PROGRAM P_Prog1
VAR

	fbKL6401 		: FB_LON_KL6401;

	fbREAD_001		: FB_READ_001_SNVT_amp;
	fbSEND_001		: FB_SEND_001_SNVT_amp;

	fbREAD_002		: FB_READ_002_SNVT_amp_mil;
	fbSEND_002		: FB_SEND_002_SNVT_amp_mil;

	fbREAD_003		: FB_READ_003_SNVT_angle;
	fbSEND_003		: FB_SEND_003_SNVT_angle;

	fbREAD_004		: FB_READ_004_SNVT_angle_vel;
	fbSEND_004		: FB_SEND_004_SNVT_angle_vel;

	fbREAD_005		: FB_READ_005_SNVT_btu_kilo;
	fbSEND_005		: FB_SEND_005_SNVT_btu_kilo;

	fbREAD_006		: FB_READ_006_SNVT_btu_mega;
	fbSEND_006		: FB_SEND_006_SNVT_btu_mega;

	fbREAD_007		: FB_READ_007_SNVT_char_ascii;
	fbSEND_007		: FB_SEND_007_SNVT_char_ascii;

	fbREAD_008		: FB_READ_008_SNVT_count;
	fbSEND_008		: FB_SEND_008_SNVT_count;

	fbREAD_009		: FB_READ_009_SNVT_count_inc;
	fbSEND_009		: FB_SEND_009_SNVT_count_inc;
(*
	fbREAD_010		: FB_READ_011_SNVT_date_day;
	fbSEND_010		: FB_SEND_002_SNVT_amp_mil;
*)

	fbREAD_011		: FB_READ_011_SNVT_date_day;
	fbSEND_011		: FB_SEND_011_SNVT_date_day;

(*
	fbREAD_012		: FB_READ_01;
	fbSEND_012		: FB_SEND_002_SNVT_amp_mil;
*)

	fbREAD_013		: FB_READ_013_SNVT_elec_kwh;
	fbSEND_013		: FB_SEND_013_SNVT_elec_kwh;

	fbREAD_014		: FB_READ_014_SNVT_elec_whr;
	fbSEND_014		: FB_SEND_014_SNVT_elec_whr;

	fbREAD_015		: FB_READ_015_SNVT_flow;
	fbSEND_015		: FB_SEND_015_SNVT_flow;

	fbREAD_016		: FB_READ_016_SNVT_flow_mil;
	fbSEND_016		: FB_SEND_016_SNVT_flow_mil;

	fbREAD_017		: FB_READ_017_SNVT_length;
	fbSEND_017		: FB_SEND_017_SNVT_length;

	fbREAD_018		: FB_READ_018_SNVT_length_kilo;
	fbSEND_018		: FB_SEND_018_SNVT_length_kilo;

	fbREAD_019		: FB_READ_019_SNVT_length_micr;
	fbSEND_019		: FB_SEND_019_SNVT_length_micr;

	fbREAD_020		: FB_READ_020_SNVT_length_mil;
	fbSEND_020		: FB_SEND_020_SNVT_length_mil;

	fbREAD_021		: FB_READ_021_SNVT_lev_cont;
	fbSEND_021		: FB_SEND_021_SNVT_lev_cont;
(*
	fbREAD_022		: FB_READ_022;
	fbSEND_022		: FB_SEND_002_SNVT_amp_mil;
*)
	fbREAD_023		: FB_READ_023_SNVT_mass;
	fbSEND_023		: FB_SEND_023_SNVT_mass;

	fbREAD_024		: FB_READ_024_SNVT_mass_kilo;
	fbSEND_024		: FB_SEND_024_SNVT_mass_kilo;

	fbREAD_025		: FB_READ_025_SNVT_mass_mega;
	fbSEND_025		: FB_SEND_025_SNVT_mass_mega;

	fbREAD_026		: FB_READ_026_SNVT_mass_mil;
	fbSEND_026		: FB_SEND_026_SNVT_mass_mil;

	fbREAD_027		: FB_READ_027_SNVT_power;
	fbSEND_027		: FB_SEND_027_SNVT_power;

	fbREAD_028		: FB_READ_028_SNVT_power_kilo;
	fbSEND_028		: FB_SEND_028_SNVT_power_kilo;

	fbREAD_029		: FB_READ_029_SNVT_ppm;
	fbSEND_029		: FB_SEND_029_SNVT_ppm;

	fbREAD_030		: FB_READ_030_SNVT_press;
	fbSEND_030		: FB_SEND_030_SNVT_press;

	fbREAD_031		: FB_READ_031_SNVT_res;
	fbSEND_031		: FB_SEND_031_SNVT_res;

END_VAR

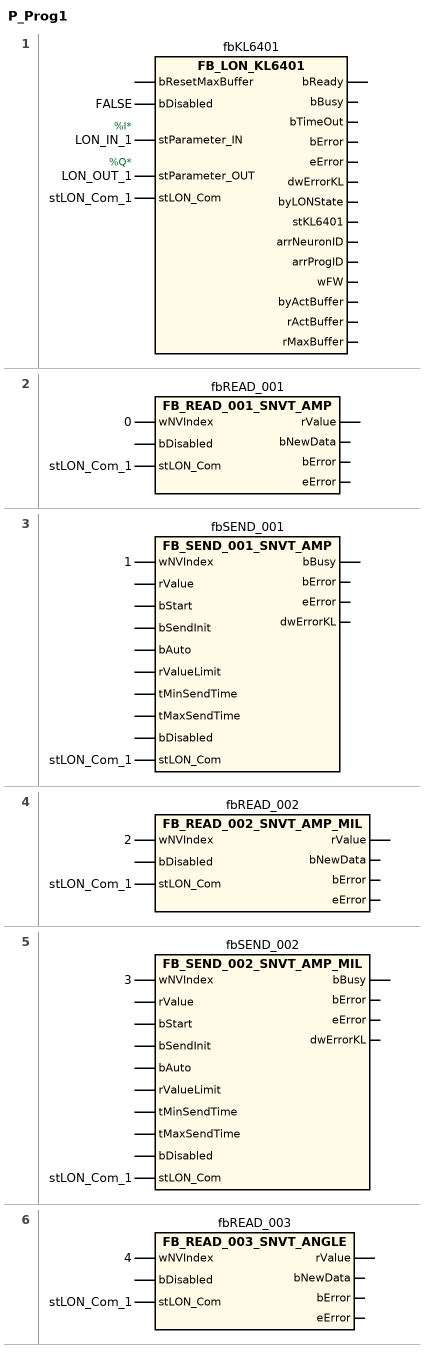
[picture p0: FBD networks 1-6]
// NETWORK 1
//   LON_IN_1: AT %I*
//   LON_OUT_1: AT %Q*
fbKL6401(
    bDisabled := FALSE,
    stParameter_IN := LON_IN_1,
    stParameter_OUT := LON_OUT_1,
    stLON_Com := stLON_Com_1); // FB_LON_KL6401

// NETWORK 2
fbREAD_001(wNVIndex := 0, stLON_Com := stLON_Com_1); // FB_READ_001_SNVT_AMP

// NETWORK 3
fbSEND_001(wNVIndex := 1, stLON_Com := stLON_Com_1); // FB_SEND_001_SNVT_AMP

// NETWORK 4
fbREAD_002(wNVIndex := 2, stLON_Com := stLON_Com_1); // FB_READ_002_SNVT_AMP_MIL

// NETWORK 5
fbSEND_002(wNVIndex := 3, stLON_Com := stLON_Com_1); // FB_SEND_002_SNVT_AMP_MIL

// NETWORK 6
fbREAD_003(wNVIndex := 4, stLON_Com := stLON_Com_1); // FB_READ_003_SNVT_ANGLE

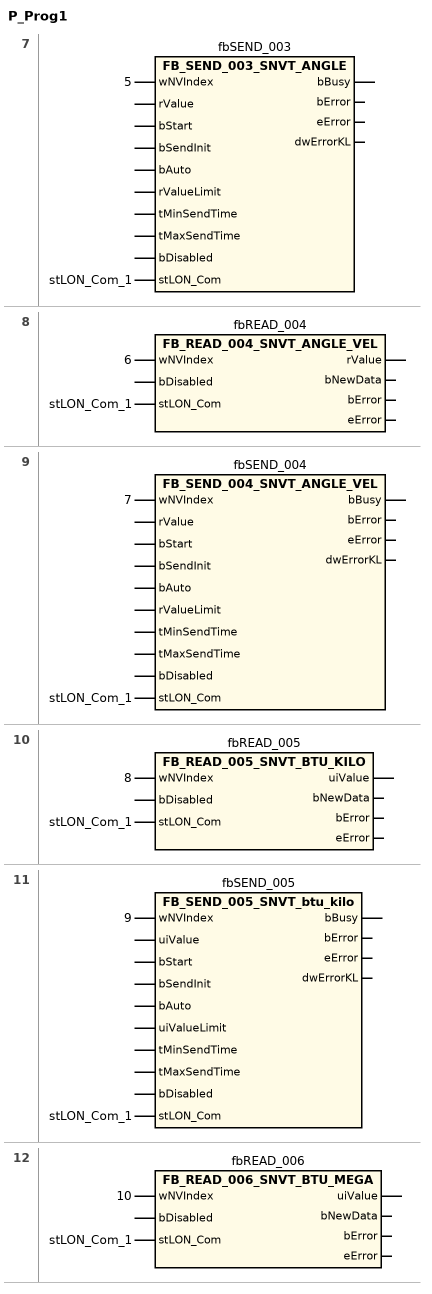
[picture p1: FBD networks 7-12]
// NETWORK 7
fbSEND_003(wNVIndex := 5, stLON_Com := stLON_Com_1); // FB_SEND_003_SNVT_ANGLE

// NETWORK 8
fbREAD_004(wNVIndex := 6, stLON_Com := stLON_Com_1); // FB_READ_004_SNVT_ANGLE_VEL

// NETWORK 9
fbSEND_004(wNVIndex := 7, stLON_Com := stLON_Com_1); // FB_SEND_004_SNVT_ANGLE_VEL

// NETWORK 10
fbREAD_005(wNVIndex := 8, stLON_Com := stLON_Com_1); // FB_READ_005_SNVT_BTU_KILO

// NETWORK 11
fbSEND_005(wNVIndex := 9, stLON_Com := stLON_Com_1); // FB_SEND_005_SNVT_btu_kilo

// NETWORK 12
fbREAD_006(wNVIndex := 10, stLON_Com := stLON_Com_1); // FB_READ_006_SNVT_BTU_MEGA

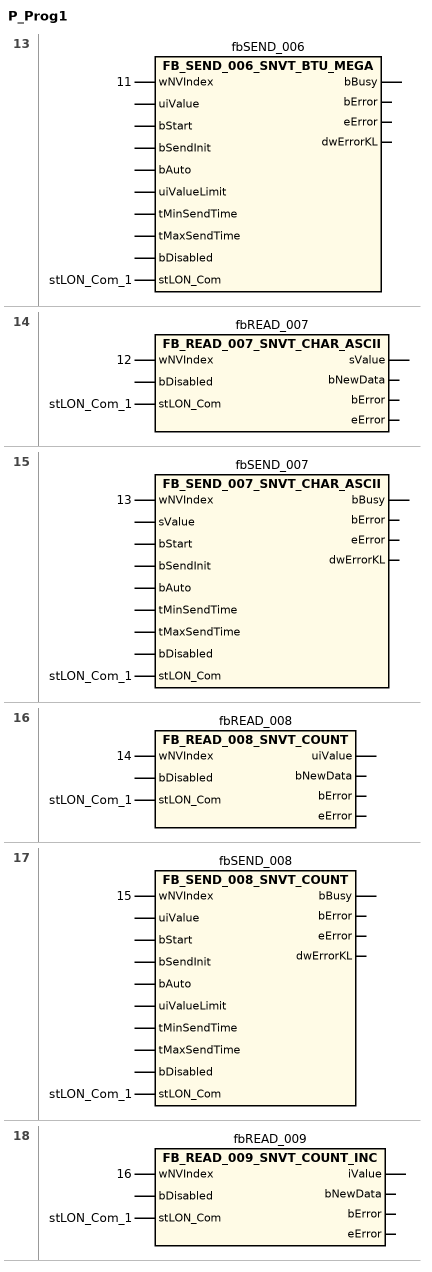
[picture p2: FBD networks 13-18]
// NETWORK 13
fbSEND_006(wNVIndex := 11, stLON_Com := stLON_Com_1); // FB_SEND_006_SNVT_BTU_MEGA

// NETWORK 14
fbREAD_007(wNVIndex := 12, stLON_Com := stLON_Com_1); // FB_READ_007_SNVT_CHAR_ASCII

// NETWORK 15
fbSEND_007(wNVIndex := 13, stLON_Com := stLON_Com_1); // FB_SEND_007_SNVT_CHAR_ASCII

// NETWORK 16
fbREAD_008(wNVIndex := 14, stLON_Com := stLON_Com_1); // FB_READ_008_SNVT_COUNT

// NETWORK 17
fbSEND_008(wNVIndex := 15, stLON_Com := stLON_Com_1); // FB_SEND_008_SNVT_COUNT

// NETWORK 18
fbREAD_009(wNVIndex := 16, stLON_Com := stLON_Com_1); // FB_READ_009_SNVT_COUNT_INC

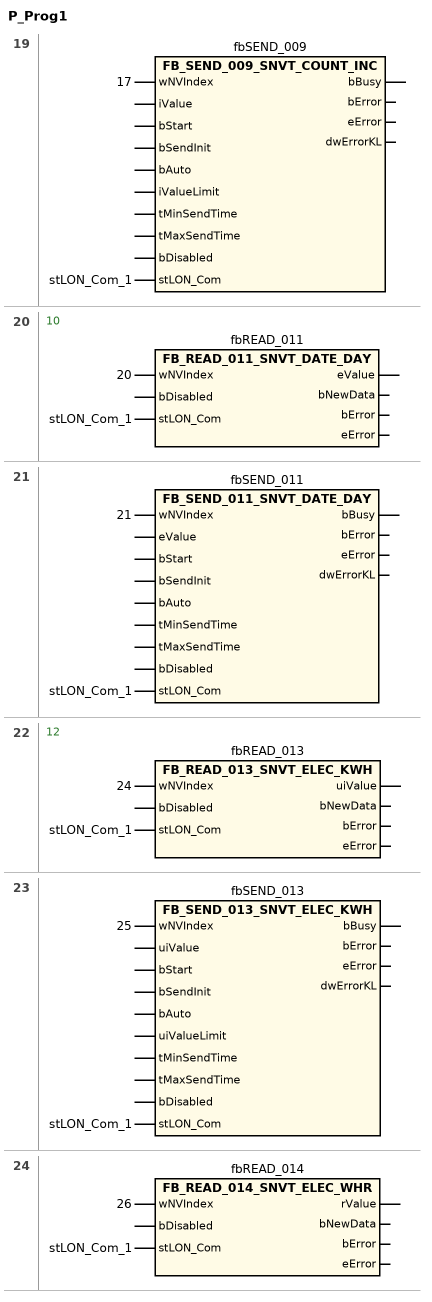
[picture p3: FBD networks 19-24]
// NETWORK 19
fbSEND_009(wNVIndex := 17, stLON_Com := stLON_Com_1); // FB_SEND_009_SNVT_COUNT_INC

// NETWORK 20
// 					10
//
//
//   fbREAD_011: fbREAD_010 : FB_READ_011_SNVT_date_day; fbSEND_010 : FB_SEND_002_SNVT_amp_mil;
fbREAD_011(wNVIndex := 20, stLON_Com := stLON_Com_1); // FB_READ_011_SNVT_DATE_DAY

// NETWORK 21
fbSEND_011(wNVIndex := 21, stLON_Com := stLON_Com_1); // FB_SEND_011_SNVT_DATE_DAY

// NETWORK 22
// 					12
//
//
//   fbREAD_013: fbREAD_012 : FB_READ_01; fbSEND_012 : FB_SEND_002_SNVT_amp_mil;
fbREAD_013(wNVIndex := 24, stLON_Com := stLON_Com_1); // FB_READ_013_SNVT_ELEC_KWH

// NETWORK 23
fbSEND_013(wNVIndex := 25, stLON_Com := stLON_Com_1); // FB_SEND_013_SNVT_ELEC_KWH

// NETWORK 24
fbREAD_014(wNVIndex := 26, stLON_Com := stLON_Com_1); // FB_READ_014_SNVT_ELEC_WHR

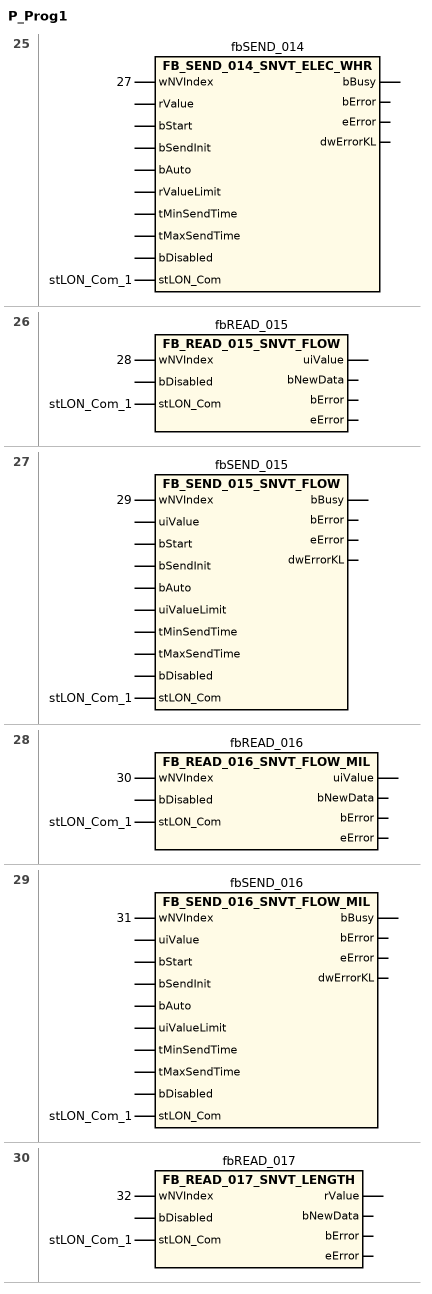
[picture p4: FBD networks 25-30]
// NETWORK 25
fbSEND_014(wNVIndex := 27, stLON_Com := stLON_Com_1); // FB_SEND_014_SNVT_ELEC_WHR

// NETWORK 26
fbREAD_015(wNVIndex := 28, stLON_Com := stLON_Com_1); // FB_READ_015_SNVT_FLOW

// NETWORK 27
fbSEND_015(wNVIndex := 29, stLON_Com := stLON_Com_1); // FB_SEND_015_SNVT_FLOW

// NETWORK 28
fbREAD_016(wNVIndex := 30, stLON_Com := stLON_Com_1); // FB_READ_016_SNVT_FLOW_MIL

// NETWORK 29
fbSEND_016(wNVIndex := 31, stLON_Com := stLON_Com_1); // FB_SEND_016_SNVT_FLOW_MIL

// NETWORK 30
fbREAD_017(wNVIndex := 32, stLON_Com := stLON_Com_1); // FB_READ_017_SNVT_LENGTH

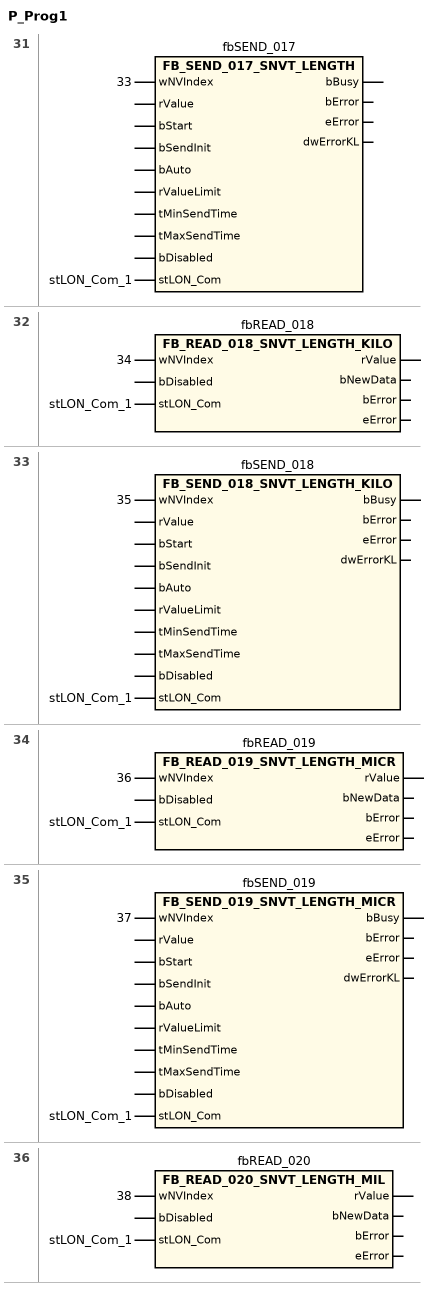
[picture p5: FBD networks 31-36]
// NETWORK 31
fbSEND_017(wNVIndex := 33, stLON_Com := stLON_Com_1); // FB_SEND_017_SNVT_LENGTH

// NETWORK 32
fbREAD_018(wNVIndex := 34, stLON_Com := stLON_Com_1); // FB_READ_018_SNVT_LENGTH_KILO

// NETWORK 33
fbSEND_018(wNVIndex := 35, stLON_Com := stLON_Com_1); // FB_SEND_018_SNVT_LENGTH_KILO

// NETWORK 34
fbREAD_019(wNVIndex := 36, stLON_Com := stLON_Com_1); // FB_READ_019_SNVT_LENGTH_MICR

// NETWORK 35
fbSEND_019(wNVIndex := 37, stLON_Com := stLON_Com_1); // FB_SEND_019_SNVT_LENGTH_MICR

// NETWORK 36
fbREAD_020(wNVIndex := 38, stLON_Com := stLON_Com_1); // FB_READ_020_SNVT_LENGTH_MIL

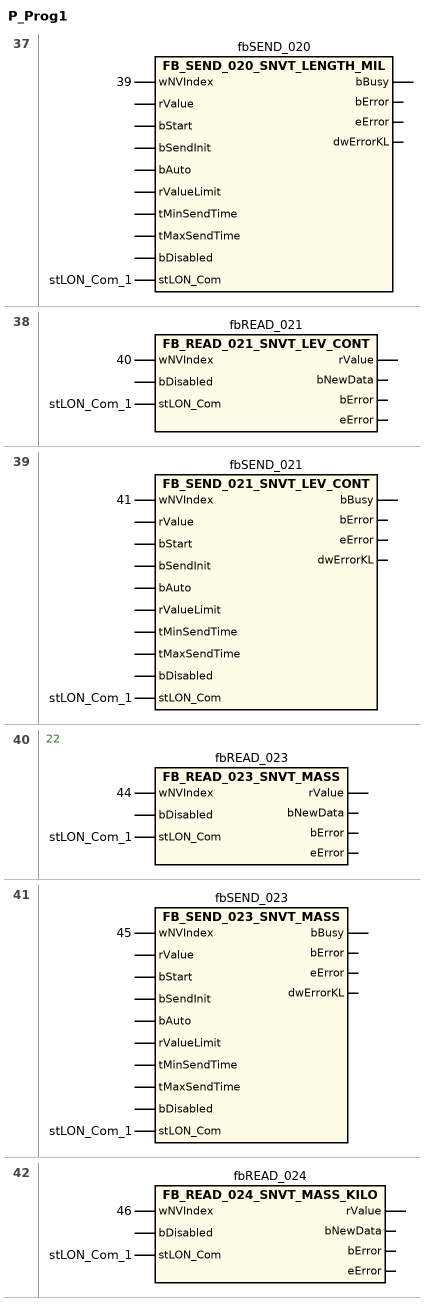
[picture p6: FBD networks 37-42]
// NETWORK 37
fbSEND_020(wNVIndex := 39, stLON_Com := stLON_Com_1); // FB_SEND_020_SNVT_LENGTH_MIL

// NETWORK 38
fbREAD_021(wNVIndex := 40, stLON_Com := stLON_Com_1); // FB_READ_021_SNVT_LEV_CONT

// NETWORK 39
fbSEND_021(wNVIndex := 41, stLON_Com := stLON_Com_1); // FB_SEND_021_SNVT_LEV_CONT

// NETWORK 40
// 					22
//
//
//   fbREAD_023: fbREAD_022 : FB_READ_022; fbSEND_022 : FB_SEND_002_SNVT_amp_mil;
fbREAD_023(wNVIndex := 44, stLON_Com := stLON_Com_1); // FB_READ_023_SNVT_MASS

// NETWORK 41
fbSEND_023(wNVIndex := 45, stLON_Com := stLON_Com_1); // FB_SEND_023_SNVT_MASS

// NETWORK 42
fbREAD_024(wNVIndex := 46, stLON_Com := stLON_Com_1); // FB_READ_024_SNVT_MASS_KILO

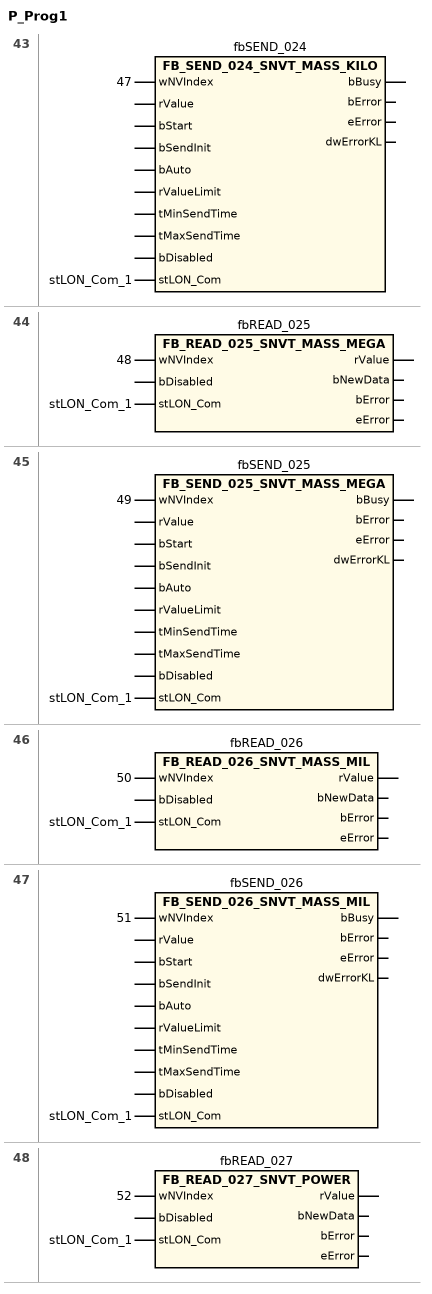
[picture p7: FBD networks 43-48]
// NETWORK 43
fbSEND_024(wNVIndex := 47, stLON_Com := stLON_Com_1); // FB_SEND_024_SNVT_MASS_KILO

// NETWORK 44
fbREAD_025(wNVIndex := 48, stLON_Com := stLON_Com_1); // FB_READ_025_SNVT_MASS_MEGA

// NETWORK 45
fbSEND_025(wNVIndex := 49, stLON_Com := stLON_Com_1); // FB_SEND_025_SNVT_MASS_MEGA

// NETWORK 46
fbREAD_026(wNVIndex := 50, stLON_Com := stLON_Com_1); // FB_READ_026_SNVT_MASS_MIL

// NETWORK 47
fbSEND_026(wNVIndex := 51, stLON_Com := stLON_Com_1); // FB_SEND_026_SNVT_MASS_MIL

// NETWORK 48
fbREAD_027(wNVIndex := 52, stLON_Com := stLON_Com_1); // FB_READ_027_SNVT_POWER

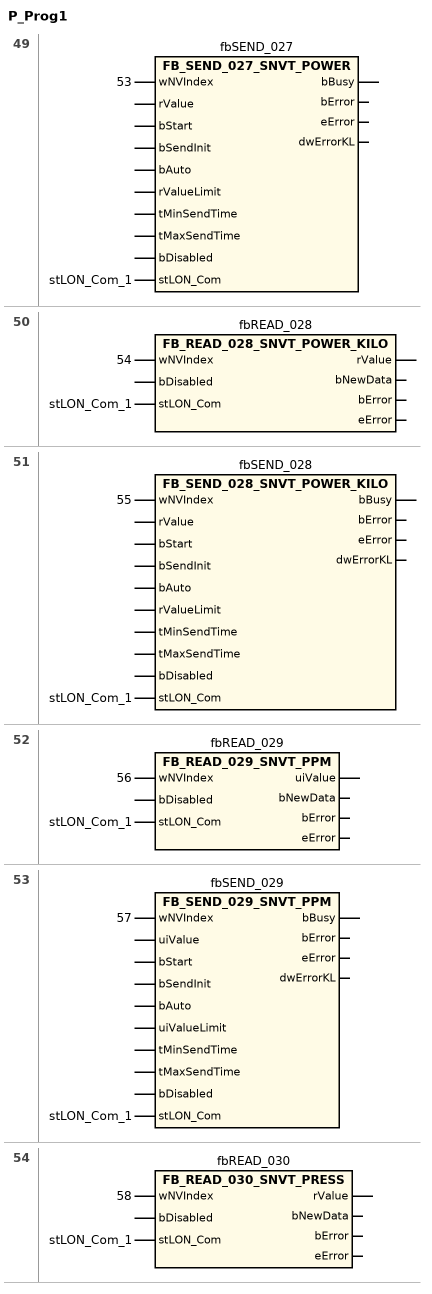
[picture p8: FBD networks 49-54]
// NETWORK 49
fbSEND_027(wNVIndex := 53, stLON_Com := stLON_Com_1); // FB_SEND_027_SNVT_POWER

// NETWORK 50
fbREAD_028(wNVIndex := 54, stLON_Com := stLON_Com_1); // FB_READ_028_SNVT_POWER_KILO

// NETWORK 51
fbSEND_028(wNVIndex := 55, stLON_Com := stLON_Com_1); // FB_SEND_028_SNVT_POWER_KILO

// NETWORK 52
fbREAD_029(wNVIndex := 56, stLON_Com := stLON_Com_1); // FB_READ_029_SNVT_PPM

// NETWORK 53
fbSEND_029(wNVIndex := 57, stLON_Com := stLON_Com_1); // FB_SEND_029_SNVT_PPM

// NETWORK 54
fbREAD_030(wNVIndex := 58, stLON_Com := stLON_Com_1); // FB_READ_030_SNVT_PRESS

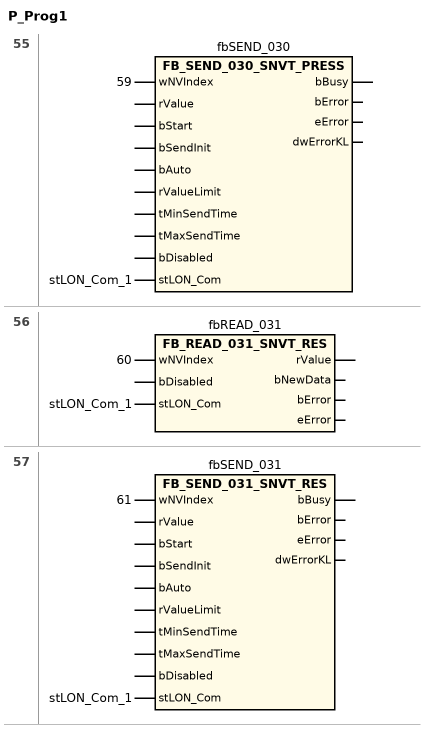
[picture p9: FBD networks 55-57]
// NETWORK 55
fbSEND_030(wNVIndex := 59, stLON_Com := stLON_Com_1); // FB_SEND_030_SNVT_PRESS

// NETWORK 56
fbREAD_031(wNVIndex := 60, stLON_Com := stLON_Com_1); // FB_READ_031_SNVT_RES

// NETWORK 57
fbSEND_031(wNVIndex := 61, stLON_Com := stLON_Com_1); // FB_SEND_031_SNVT_RES

END_PROGRAM
